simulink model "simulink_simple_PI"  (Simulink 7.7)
settings: Solver=ode15s  StartTime=0.0  StopTime=24  RelTol=1e-3
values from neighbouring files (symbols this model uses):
  A = [((-UAfr)/mCpf) (UAfr/mCpf) 0; (UAfr/mCpr) ((-UAro-UAfr)/mCpr) 0; 0 0 0]    [simplemodel.m]
  B = [1/mCpf 0 0 ; 0 1/mCpr (UAro/mCpr); 0 1 0]    [simplemodel.m]
  C = [1 0 0; 0 1 0; 0 0 1]    [simplemodel.m]
  D = [0 0 0 ; 0 0 0; 0 0 0]    [simplemodel.m]
  init = [Tf Tr E]    [simplemodel.m]
  qhf = 0    [simplemodel.m]
  qhr = 4000*60*60    (= 14400000)    [simplemodel.m]
  Tmax = 293    [simplemodel.m]
  Tmin = 283    [simplemodel.m]
  To = 273+0    (= 273)    [simplemodel.m]
  Trset = 293    [simplemodel.m]
libraries: simulink x1

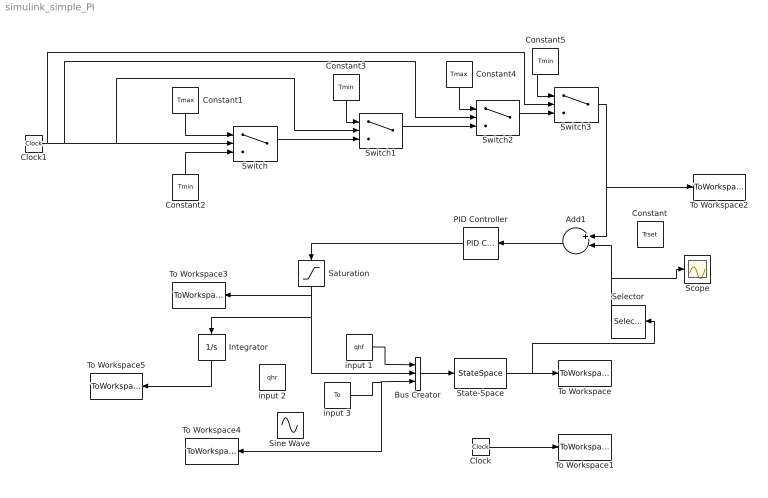
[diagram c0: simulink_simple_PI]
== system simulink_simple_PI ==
  Add1 : Sum  Inputs=+-
  Bus Creator : BusCreator  Inputs=3
  Clock : Clock
  Clock1 : Clock
  Constant : Constant  Value=Trset
  Constant1 : Constant  Value=Tmax
  Constant2 : Constant  Value=Tmin
  Constant3 : Constant  Value=Tmin
  Constant4 : Constant  Value=Tmax
  Constant5 : Constant  Value=Tmin
  Integrator : Integrator
  PID Controller : simulink/Continuous/PID Controller  SystemSampleTime=-1  Controller=PI  TimeDomain=Continuous-time  SampleTime=1  IntegratorMethod=Forward Euler  FilterMethod=Forward Euler  Form=Parallel  P=7032008.284*4  I=175800207.1  D=0  N=100  InitialConditionSource=internal  InitialConditionForIntegrator=0  InitialConditionForFilter=0  ExternalReset=none  LimitOutput=on  UpperSaturationLimit=4000*60*60  LowerSaturationLimit=0  LinearizeAsGain=off  AntiWindupMode=clamping  Kb=1  TrackingMode=off  Kt=1  PParamMin=[]  PParamMax=[]  IParamMin=[]  IParamMax=[]  DParamMin=[]  DParamMax=[]  NParamMin=[]  NParamMax=[]  KbParamMin=[]  KbParamMax=[]  KtParamMin=[]  KtParamMax=[]  POutMin=[]  POutMax=[]  IOutMin=[]  IOutMax=[]  DOutMin=[]  DOutMax=[]  NOutMin=[]  NOutMax=[]  KbOutMin=[]  KbOutMax=[]  KtOutMin=[]  KtOutMax=[]  IntegratorOutMin=[]  IntegratorOutMax=[]  FilterOutMin=[]  FilterOutMax=[]  SumOutMin=[]  SumOutMax=[]  SumI1OutMin=[]  SumI1OutMax=[]  SumI2OutMin=[]  SumI2OutMax=[]  SumI3OutMin=[]  SumI3OutMax=[]  SumDOutMin=[]  SumDOutMax=[]  SaturationOutMin=[]  SaturationOutMax=[]  IntegratorContinuousStateAttributes=''  IntegratorStateMustResolveToSignalObject=off  IntegratorRTWStateStorageClass=Auto  FilterContinuousStateAttributes=''  FilterStateMustResolveToSignalObject=off  FilterRTWStateStorageClass=Auto
  Saturation : Saturate  UpperLimit=4000*60*60  LowerLimit=0
  Scope : Scope
  Selector : Selector  InputPortWidth=3  IndexOptions=Index vector (dialog)  Indices=2  OutputSizes=1
  Sine Wave : Sin  Amplitude=10  Bias=273  Frequency=(2*pi())/24  Phase=-pi()/2  SampleTime=0
  State-Space : StateSpace  A=A  B=B  C=C  D=D  X0=init
  Switch : Switch  Threshold=3.5
  Switch1 : Switch  Threshold=9.6
  Switch2 : Switch  Threshold=13.94
  Switch3 : Switch  Threshold=19.2
  To Workspace : ToWorkspace  VariableName=simout  SampleTime=-1  SaveFormat=Array
  To Workspace1 : ToWorkspace  VariableName=time  SampleTime=-1  SaveFormat=Array
  To Workspace2 : ToWorkspace  VariableName=Set_out  SampleTime=-1  SaveFormat=Array
  To Workspace3 : ToWorkspace  VariableName=Qhr  SampleTime=-1  SaveFormat=Array
  To Workspace4 : ToWorkspace  VariableName=To_out  SampleTime=-1  SaveFormat=Array
  To Workspace5 : ToWorkspace  VariableName=E_out  SampleTime=-1  SaveFormat=Array
  input 1 : Constant  Value=qhf
  input 2 : Constant  Value=qhr
  input 3 : Constant  Value=To
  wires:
  Bus Creator/1 -> State-Space/1
  State-Space/1 -> To Workspace/1, Selector/1
  Clock/1 -> To Workspace1/1
  Selector/1 -> Add1/2, Scope/1
  Add1/1 -> PID Controller/1
  input 1/1 -> Bus Creator/1
  Constant1/1 -> Switch/1
  Constant2/1 -> Switch/3
  Clock1/1 -> Switch/2, Switch1/2, Switch2/2, Switch3/2
  Switch/1 -> Switch1/3
  Constant3/1 -> Switch1/1
  Switch1/1 -> Switch2/3
  Constant4/1 -> Switch2/1
  PID Controller/1 -> Saturation/1
  Saturation/1 -> To Workspace3/1, Bus Creator/2, Integrator/1
  Switch2/1 -> Switch3/3
  Switch3/1 -> To Workspace2/1, Add1/1
  Constant5/1 -> Switch3/1
  Integrator/1 -> To Workspace5/1
  input 3/1 -> Bus Creator/3, To Workspace4/1
